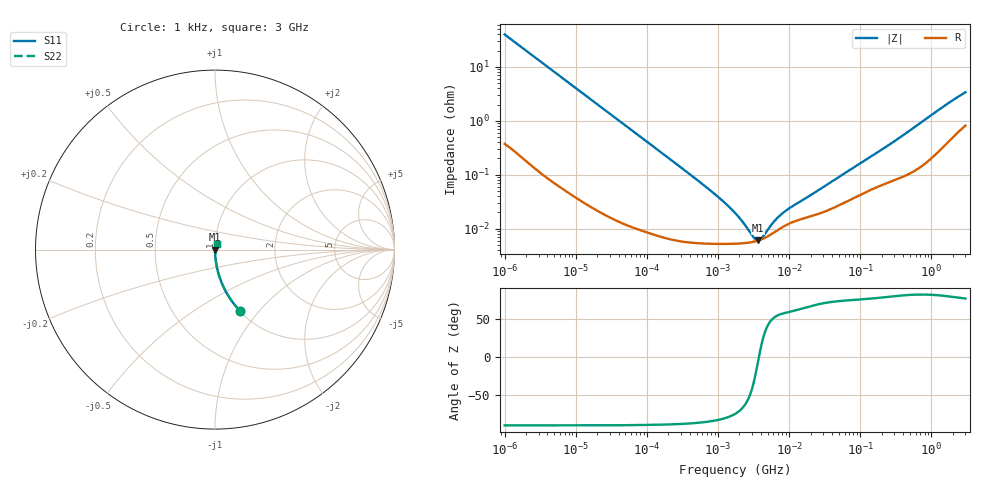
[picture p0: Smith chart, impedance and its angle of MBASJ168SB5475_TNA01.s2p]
! MBASJ168SB5475_TNA01  S-PARAMETER MODEL  ( Standard Model )
! Model Generated by TAIYO YUDEN Corporation (http://www.ty-top.com)
! Version 1.0
! TAIYO YUDEN Control No. 220601
! Copyright(c) 2012 TAIYO YUDEN CO.,LTD. All Rights Reserved.
! Product Description (link to TY-COMPAS)
! https://ds.yuden.co.jp/TYCOMPAS/or/detail?pn=MBASJ168SB5475KTNA01&u=M
! Products Name : Multilayer Ceramic Capacitors
! Characteristics :
!  Capacitance : 4.7 [uF] , Rated Voltage : 6.3 [V] , TCC : X5R
!  Case Size : 1.6 x 0.8 / 0.063 x 0.031 [mm/inch] , Thickness : 0.8 / 0.031 [mm/inch]
!  (Conditions: Temperature = 25 [degC] , DC Bias Voltage = 0 [V])
! External Node Assignments :
!  1  o---| |---o  2
! GND o---------o GND
! Frequency Range : 1kHz  -  3GHz  [ 401 STEP ]
# MHZ S RI R 50
! Freq[MHz].  S11 Real  S11 Imag  S21 Real  S21 Imag  S12 Real  S12 Imag  S22 Real  S22 Imag
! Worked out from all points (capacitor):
!   401 points, 1 kHz to 3 GHz, reference 50 ohm
!   read as one part in series: C = 3.97 uF near 1.077 kHz
!   lowest |Z| = 6.02 mohm at 3.651 MHz (marker M1)
!   series resonance near 3.76 MHz, so ESL is about 450 pH
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0.001  0.14 -0.3424  0.86 0.3424  0.86 0.3424  0.14 -0.3424
0.001685  0.0554 -0.2243  0.9446 0.2243  0.9446 0.2243  0.0554 -0.2243
0.00306  0.0181 -0.129  0.9819 0.129  0.9819 0.129  0.0181 -0.129
0.005768  0.00547 -0.0695  0.9945 0.0695  0.9945 0.0695  0.00547 -0.0695
0.01216  0.00143 -0.0333  0.9986 0.0333  0.9986 0.0333  0.00143 -0.0333
0.033275  0.0003 -0.0122  0.9997 0.0122  0.9997 0.0122  0.0003 -0.0122
0.147855  7.96e-05 -0.00277  0.9999 0.00277  0.9999 0.00277  7.96e-05 -0.00277
0.791611  5.24e-05 -0.000499  0.9999 0.000499  0.9999 0.000499  5.24e-05 -0.000499
1.238299  5.2e-05 -0.000298  0.9999 0.000298  0.9999 0.000298  5.2e-05 -0.000298
1.732051  5.23e-05 -0.000189  0.9999 0.000189  0.9999 0.000189  5.23e-05 -0.000189
2.422679  5.39e-05 -0.0001  0.9999 0.0001  0.9999 0.0001  5.39e-05 -0.0001
2.610246  5.45e-05 -8.26e-05  0.9999 8.26e-05  0.9999 8.26e-05  5.45e-05 -8.26e-05
2.812335  5.53e-05 -6.52e-05  0.9999 6.52e-05  0.9999 6.52e-05  5.53e-05 -6.52e-05
3.651041  5.99e-05 -6.43e-06  0.9999 6.43e-06  0.9999 6.43e-06  5.99e-05 -6.43e-06
4.739869  6.91e-05 5.06e-05  0.9999 -5.06e-05  0.9999 -5.06e-05  6.91e-05 5.06e-05
5.106836  7.3e-05 6.67e-05  0.9999 -6.67e-05  0.9999 -6.67e-05  7.3e-05 6.67e-05
6.881678  9.34e-05 0.000129  0.9999 -0.000129  0.9999 -0.000129  9.34e-05 0.000129
8.606987  0.000112 0.000173  0.9999 -0.000173  0.9999 -0.000173  0.000112 0.000173
21.06097  0.000172 0.000399  0.9998 -0.000399  0.9998 -0.000399  0.000172 0.000399
256.0921  0.000737 0.00353  0.9993 -0.00353  0.9993 -0.00353  0.000737 0.00353
1591.635  0.004 0.0192  0.996 -0.0192  0.996 -0.0192  0.004 0.0192
3000  0.0091 0.0323  0.9909 -0.0323  0.9909 -0.0323  0.0091 0.0323
